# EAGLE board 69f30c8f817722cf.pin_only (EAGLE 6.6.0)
REV: A

Size 34.29 x 24.13 mm. Coordinates in mm from the lower left corner, seen from the top.
Outline: 34.29,2.54 34.29,21.59 arc90 31.75,24.13 2.54,24.13 arc90 0,21.59 0,2.54 arc90 2.54,0 31.75,0 arc90 34.29,2.54
Copper layers (1*16): Top 0.035mm / dielectric 1.5mm / Bottom 0.035mm
Design rules "adafruit": minimum track width 8mil, minimum drill 15.5mil, track to track 8mil, track to pad 8mil, pad to pad 8mil, via to via 8mil, smd to smd 8mil, copper to edge 10mil, drill to drill 8mil, minimum pad ring 10mil, minimum via ring 8mil, stop-mask expansion 2mil, vias tented up to drill 20mil, thermal gap 10mil
tRestrict: area 18.9,2.1 to 19.1,2.6; area 17.6,2.1 to 17.8,2.7; area 16.4,2.1 to 16.6,2.7; area 16.7,3.8 to 17.3,3.9

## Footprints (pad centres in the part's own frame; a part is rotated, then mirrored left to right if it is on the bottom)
FIDUCIAL_1MM = smd 1 x 1: 1 0,0
MOUNTINGHOLE_2.5_PLATED = drill 2.5 pad 3.2: P$1 0,0
2X05_1.27MM_BOX_POSTS = smd 0.76 x 2.6: 1 -2.54,-2.15; 2 -2.54,2.15; 3 -1.27,-2.15; 4 -1.27,2.15; 5 0,-2.15; 6 0,2.15; 7 1.27,-2.15; 8 1.27,2.15; 9 2.54,-2.15; 10 2.54,2.15 | hole 1: -1.905,0; 1.905,0
2X10_SMT_FEMALE = smd 1.02 x 5: 1 -11.43,-3; 2 -11.43,3; 3 -8.89,-3; 4 -8.89,3; 5 -6.35,-3; 6 -6.35,3; 7 -3.81,-3; 8 -3.81,3; 9 -1.27,-3; 10 -1.27,3; 11 1.27,-3; 12 1.27,3; 13 3.81,-3; 14 3.81,3; 15 6.35,-3; 16 6.35,3; 17 8.89,-3; 18 8.89,3; 19 11.43,-3; 20 11.43,3

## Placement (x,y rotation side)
FID1  FIDUCIAL""  [FIDUCIAL_1MM]  32,20.57 0 top
FID2  FIDUCIAL""  [FIDUCIAL_1MM]  2.54,6.86 0 top
U$3  [ADAFRUIT_5MM]  5.42,2.67 0 top
U$4  [PCBFEAT-REV-056]  7.44,1.61 0 top
U$5  MOUNTINGHOLE2.5  [MOUNTINGHOLE_2.5_PLATED]  2.54,2.54 0 top
U$6  MOUNTINGHOLE2.5  [MOUNTINGHOLE_2.5_PLATED]  31.75,2.54 0 top
X1  20317  [2X05_1.27MM_BOX_POSTS]  17.14,4.45 0 top
X2  03587  [2X10_SMT_FEMALE]  17.14,17.78 0 top

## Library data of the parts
FID1 FID2 U$5 U$6 = microbuilder; BOM: EXCLUDE
U$3 U$4 X1 X2 = microbuilder

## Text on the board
tPlace: 2x10 0.1" | CORTEX SWD Adapter | 2x5 0.05"
bPlace: JTAG PINOUT | SWD PINOUT | NC | VREF | SWDIO/TMS | VCC | SWDCLK/TCK | GND | GND | NC | GND | TDI | SWO/TDO | GND | GND | TMS | NC/TDI | KEY | GND | TCK | nRESET | GND | GND | NC | GND | TDO | GND | nRESET | GND | NC | GND | NC

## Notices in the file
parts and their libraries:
microbuilder: This work is placed in the public domain, and may be freely used for commercial and non-commercial work with the following conditions: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
